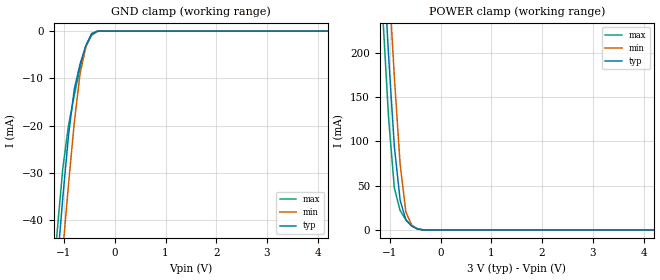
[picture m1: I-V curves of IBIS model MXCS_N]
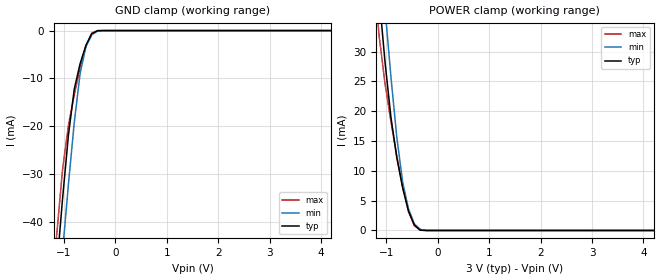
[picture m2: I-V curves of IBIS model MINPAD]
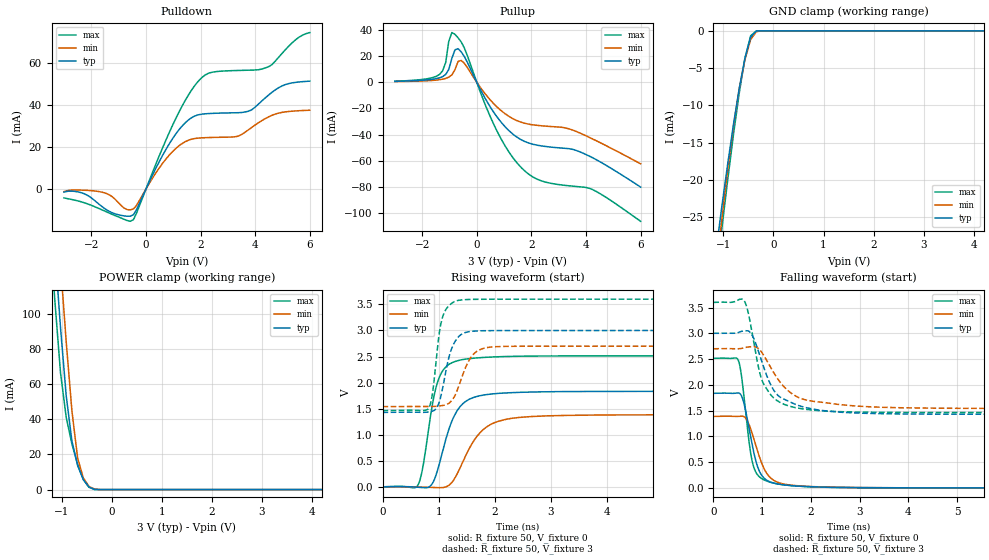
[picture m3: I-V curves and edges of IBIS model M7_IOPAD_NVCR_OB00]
| Created by SiliconSmart  O-2018.09-SP2-3
[IBIS Ver]   4.0
[File Name]   as3204wa_rev1p4.ibs
[File Rev]   1.4
[Date]   Thursday Mar 21 2024
|[Source]   Avalanche Team
|[Notes]   Generated IBIS models from Silicon Smart
|[Rev 1.0]  Initial Release based on extracted netlist
|   Characterization
|[Rev 1.1]  Update the drive strength table for 3V
|[Rev 1.2]  Recharacterization of MIOPAD with Hspice run in high accuracy mode
|[Rev 1.3]  Recharacterization with Hspice to align with datasheet parameter
|[Rev 1.4]  Update the pin to the package pinout assignment
|[Disclaimer]   THE MODEL LIBRARIES ARE PROVIDED AS IS.
|[Copyright]   Copyright 2019, Avalanche Technology., All Rights Reserved
[Component]   AS30xx204_WSON
[Manufacturer] Avalanche Technology
| CONTENT :
| This file contains IBIS MODEL for PSRAM device
| AS3001204 AS3004204 AS3008204 AS3016204
| USAGE :
| The models are derived for the 2.7V to 3.6V I/O Operation.
| Temperatures for model generation: typ: 25, max: -40, min: 105
| Voltages : typ: 3.0V, min: 2.7V, max: 3.6V
| PACKAGES SUPPORTED :
| 8-pad WSON (5.0mm x 6.0mm)
| VERIFICATION
| Errors  : 0
| Warnings: 30
| All warnings due to non-monotonic data:
[Package]
|variable   typ   min   max
R_pkg   8.90E-04   8.89E-04  8.91E-04
L_pkg   1.185E-09  1.18E-09  1.19E-09
C_pkg   2.30E-13   2.21E-13  2.39E-13
[Pin]   signal_name   model_name   R_pin   L_pin   C_pin
1   CS#   MXCS_N   1.05E-01  1.35E-09  9.16E-14
2   SO   MIOPAD   1.05E-01  1.35E-09  9.16E-14
3   WP#   MIOPAD   1.05E-01  1.35E-09  9.16E-14
5   SI   MIOPAD   3.75E-02  3.89E-10  4.24E-14
6   CLK   MINPAD   3.75E-02  3.89E-10  4.24E-14
7   IO_3   MIOPAD   3.75E-02  3.89E-10  4.24E-14
4   VSS   GND   NA   NA   NA
8   VCC   POWER   NA   NA   NA
[Model Selector] MIOPAD
| Model Description
M0_IOPAD_NVCR_OB07   15 Ohms drv strength
M1_IOPAD_NVCR_OB06   20 Ohms drv strength
M2_IOPAD_NVCR_OB05   40 Ohms drv strength
M3_IOPAD_NVCR_OB04   35 Ohms drv strength
M4_IOPAD_NVCR_OB03   45 Ohms drv strength
M5_IOPAD_NVCR_OB02   60 Ohms drv strength
M6_IOPAD_NVCR_OB01   75 Ohms drv strength
M7_IOPAD_NVCR_OB00   35 Ohms drv strength
| Models and submodels in the file (10): MXCS_N (Input), MINPAD (Input), M7_IOPAD_NVCR_OB00 (I/O), M3_IOPAD_NVCR_OB04 (I/O), M5_IOPAD_NVCR_OB02 (I/O), M1_IOPAD_NVCR_OB06 (I/O), M6_IOPAD_NVCR_OB01 (I/O), M2_IOPAD_NVCR_OB05 (I/O), M4_IOPAD_NVCR_OB03 (I/O), M0_IOPAD_NVCR_OB07 (I/O)
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| XCS_N
[Model] MXCS_N
Model_type Input
Enable   Active-High
Vinl  =  0.9
Vinh  =  2.1
| Capacitance  typ   min   max
C_comp   3.070316e-12   2.808436e-12   3.350457e-12
| Variables   typ   min   max
[GND Clamp Reference]   0   0   0
[POWER Clamp Reference]   3   2.7   3.6
[Pulldown Reference]   0   0   0
[Pullup Reference]   3   2.7   3.6
[Temperature Range]   25   105   -40
[Voltage Range]   3   2.7   3.6
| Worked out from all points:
|   GND clamp passes 1 mA (typ) near -0.47 V on its own axis
|   POWER clamp passes 1 mA (typ) near -0.45 V on its own axis
[GND Clamp]
| Voltage   I(typ)   I(min)   I(max)
-3V       -315.1mA   -321.8mA   -312.6mA
-1.138V   -50.1mA    -61.4mA    -42.93mA
-1.024V   -35.38mA   -46.59mA   -29.17mA
-910.3mV  -22.01mA   -32.38mA   -19.91mA
-796.6mV  -12.29mA   -19.34mA   -13.52mA
-682.8mV  -6.93mA    -8.967mA   -7.783mA
-569mV    -3.073mA   -3.363mA   -3.169mA
-455.2mV  -632.4uA   -876.6uA   -499.8uA
-341.4mV  -24.5uA    -77.16uA   -7.616uA
-227.6mV  -421.5nA   -3.518uA   -35.99nA
6V        0A         0A         0A
[POWER Clamp]
| Voltage   I(typ)   I(min)   I(max)
-3V       2.46A      2.545A     2.395A
-1.138V   315.5mA    408mA      242.2mA
-1.024V   197.2mA    287.4mA    127mA
-910.3mV  94.22mA    172.8mA    47.4mA
-796.6mV  33.73mA    74.33mA    21.95mA
-682.8mV  11.27mA    20.05mA    11.43mA
-569mV    4.378mA    5.6mA      4.484mA
-455.2mV  1.088mA    1.361mA    987.1uA
-227.6mV  835.3nA    9.424uA    241.1nA
6V        0A         0A         0A
| INPAD
[Model] MINPAD
Model_type Input
Enable   Active-High
Vinl  =  0.9
Vinh  =  2.1
| Capacitance  typ   min   max
C_comp   2.706389e-12   2.515315e-12   2.914212e-12
| Variables   typ   min   max
[GND Clamp Reference]   0   0   0
[POWER Clamp Reference]   3   2.7   3.6
[Pulldown Reference]   0   0   0
[Pullup Reference]   3   2.7   3.6
[Temperature Range]   25   105   -40
[Voltage Range]   3   2.7   3.6
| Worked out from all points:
|   GND clamp passes 1 mA (typ) near -0.47 V on its own axis
|   POWER clamp passes 1 mA (typ) near -0.46 V on its own axis
[GND Clamp]
| Voltage   I(typ)   I(min)   I(max)
-3V       -312.9mA   -319.5mA   -311mA
-1.138V   -49.77mA   -60.97mA   -42.7mA
-1.024V   -35.15mA   -46.28mA   -29.02mA
-910.3mV  -21.89mA   -32.17mA   -19.81mA
-796.6mV  -12.24mA   -19.23mA   -13.45mA
-682.8mV  -6.904mA   -8.93mA    -7.747mA
-569mV    -3.064mA   -3.355mA   -3.158mA
-455.2mV  -631.5uA   -875.4uA   -499.1uA
-341.4mV  -24.5uA    -77.14uA   -7.616uA
-227.6mV  -421.5nA   -3.518uA   -35.99nA
6V        0A         0A         0A
[POWER Clamp]
| Voltage   I(typ)   I(min)   I(max)
-3V       249.7mA    259.7mA    242mA
-1.252V   50.97mA    61.19mA    43.36mA
-1.138V   39.14mA    48.99mA    32.5mA
-1.024V   28.15mA    37.13mA    24.58mA
-910.3mV  19.01mA    25.79mA    18.3mA
-796.6mV  12.24mA    15.66mA    12.48mA
-682.8mV  7.193mA    8.146mA    7.285mA
-569mV    3.26mA     3.629mA    3.179mA
-455.2mV  915uA      1.117mA    809.1uA
-341.4mV  55.3uA     196.8uA    44.86uA
-113.8mV  7.997nA    354.9nA    881.5pA
6V        0A         0A         0A
[Model] M7_IOPAD_NVCR_OB00
Model_type I/O
Enable   Active-High
Vinl  =  0.9
Vinh  =  2.1
Vmeas =  1.5
Cref  =  30e-12
| Capacitance  typ   min   max
C_comp   3.872127e-12   3.590660e-12   4.176448e-12
| Variables   typ   min   max
[GND Clamp Reference]   0   0   0
[POWER Clamp Reference]   3   2.7   3.6
[Pulldown Reference]   0   0   0
[Pullup Reference]   3   2.7   3.6
[Temperature Range]   25   105   -40
[Voltage Range]   3   2.7   3.6
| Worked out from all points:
|   slope of the pulldown table from 0 to 0.45 V, typ, clamps not added: 37.1 ohm
|   slope of the pullup table from 0 to 0.45 V, typ, clamps not added: 25.9 ohm
|   GND clamp passes 1 mA (typ) near -0.46 V on its own axis
|   POWER clamp passes 1 mA (typ) near -0.42 V on its own axis
|   falling waveform, R_fixture 50, V_fixture 0: 20-80 % time 256ps typ, 321ps min, 201ps max; typ from 1.83 V to 0 V
|   falling waveform, R_fixture 50, V_fixture 3: 20-80 % time 490ps typ, 612ps min, 350ps max; typ from 3 V to 1.43 V
|   rising waveform, R_fixture 50, V_fixture 0: 20-80 % time 339ps typ, 461ps min, 243ps max; typ from 0 V to 1.83 V
|   rising waveform, R_fixture 50, V_fixture 3: 20-80 % time 204ps typ, 266ps min, 147ps max; typ from 1.43 V to 3 V
[GND Clamp]
| Voltage   I(typ)   I(min)   I(max)
-3V       -145.9mA   -151.9mA   -144.2mA
-1.138V   -29.07mA   -31.55mA   -32.68mA
-1.024V   -23.24mA   -24.83mA   -26.15mA
-910.3mV  -17.69mA   -18.46mA   -19.83mA
-796.6mV  -12.47mA   -12.67mA   -13.82mA
-682.8mV  -7.718mA   -7.754mA   -8.316mA
-569mV    -3.663mA   -3.867mA   -3.675mA
-455.2mV  -839.2uA   -1.152mA   -666.1uA
-341.4mV  -35.63uA   -111.1uA   -11.17uA
-113.8mV  -8.642nA   -188.3nA   -1.888nA
6V        0A         0A         0A
[POWER Clamp]
| Voltage   I(typ)   I(min)   I(max)
-3V       949.8mA    984.2mA    923.5mA
-1.252V   183.6mA    221.4mA    154mA
-1.138V   136.7mA    174.2mA    107.6mA
-1.024V   92.09mA    128.1mA    66.35mA
-910.3mV  53.33mA    83.97mA    41.06mA
-796.6mV  27.72mA    44.75mA    25.94mA
-682.8mV  13.75mA    18.06mA    14.29mA
-569mV    5.664mA    6.605mA    5.738mA
-455.2mV  1.446mA    1.789mA    1.305mA
-341.4mV  77.09uA    287.6uA    62.73uA
-227.6mV  1.148uA    12.92uA    332nA
6V        0A         0A         0A
[Pulldown]
| Voltage   I(typ)   I(min)   I(max)
-3V       -1.433mA   -1.188mA   -4.157mA
-2.276V   -2.108mA   -517.7uA   -6.425mA
-1.593V   -8.473mA   -1.507mA   -9.973mA
-455.2mV  -12.21mA   -9.42mA    -14.49mA
931mV     23.15mA    17.28mA    29.13mA
1.448V    31.69mA    22.63mA    42.45mA
1.966V    35.52mA    24.35mA    52.07mA
2.483V    36.1mA     24.62mA    55.8mA
3.745V    37.06mA    28.17mA    56.63mA
4.49V     44.79mA    34.41mA    58.29mA
5.11V     49.81mA    36.8mA     66.46mA
6V        51.42mA    37.57mA    74.56mA
[Pullup]
| Voltage   I(typ)   I(min)   I(max)
-3V       653.5uA    487.7uA    766.8uA
-1.366V   3.311mA    1.902mA    5.899mA
-1.138V   5.906mA    2.886mA    14.98mA
-1.024V   9.73mA     3.87mA     31.24mA
-910.3mV  18.3mA     5.605mA    37.88mA
-796.6mV  24.73mA    9.674mA    36.53mA
-569mV    23.14mA    16.61mA    30.71mA
620.7mV   -22.92mA   -16.38mA   -32.1mA
1.655V    -44.22mA   -30.74mA   -65.72mA
2.379V    -48.66mA   -33.29mA   -75.39mA
3.745V    -52.9mA    -38.5mA    -79.8mA
6V        -80.07mA   -62.32mA   -106.2mA
[Ramp]
dV/dt_r   1.10101/0.339017n  0.831927/0.461224n  1.50845/0.242789n
dV/dt_f   0.94313/0.490001n  0.695697/0.612195n  1.28285/0.34977n
R_load = 50
[Falling Waveform]
R_fixture = 50
V_fixture = 0
V_fixture_min = 0
V_fixture_max = 0
| Time   V(typ)   V(min)   V(max)
0s        1.835V     1.387V     2.514V
508.1ps   1.842V     1.388V     2.484V
563ps     1.81V      1.393V     2.266V
628.4ps   1.639V     1.383V     1.772V
754.2ps   1.042V     1.175V     742mV
850.8ps   600.9mV    886.9mV    345.7mV
956.7ps   299.5mV    569.6mV    204.1mV
1.112ns   137.8mV    259.2mV    126.2mV
1.514ns   51.15mV    62.52mV    51.11mV
21.88ns   622.8nV    711.5nV    10.89uV
[Falling Waveform]
R_fixture = 50
V_fixture = 3
V_fixture_min = 2.7
V_fixture_max = 3.6
| Time   V(typ)   V(min)   V(max)
0s        3V         2.7V       3.6V
624.2ps   3.048V     2.717V     3.642V
788.3ps   2.977V     2.741V     3.046V
963.4ps   2.539V     2.667V     2.19V
1.115ns   2.134V     2.441V     1.888V
1.308ns   1.809V     2.134V     1.693V
1.506ns   1.7V       1.909V     1.603V
2.036ns   1.53V      1.682V     1.509V
4.777ns   1.43V      1.545V     1.463V
21.88ns   1.428V     1.54V      1.462V
[Rising Waveform]
R_fixture = 50
V_fixture = 0
V_fixture_min = 0
V_fixture_max = 0
| Time   V(typ)   V(min)   V(max)
0s        414.5nV    452.2nV    10.8uV
619.8ps   -611.3uV   5.242mV    21.45mV
717.4ps   -8.991mV   2.623mV    378.7mV
871ps     45.71mV    -3.239mV   1.477V
1.013ns   453.4mV    -9.161mV   2.11V
1.262ns   1.331V     129.2mV    2.395V
1.571ns   1.696V     791.7mV    2.465V
2.006ns   1.791V     1.241V     2.495V
2.928ns   1.827V     1.365V     2.512V
21.88ns   1.835V     1.387V     2.514V
[Rising Waveform]
R_fixture = 50
V_fixture = 3
V_fixture_min = 2.7
V_fixture_max = 3.6
| Time   V(typ)   V(min)   V(max)
0s        1.428V     1.54V      1.462V
810.7ps   1.438V     1.544V     1.497V
887.5ps   1.456V     1.544V     1.779V
1.003ns   1.607V     1.552V     2.894V
1.068ns   1.883V     1.562V     3.253V
1.21ns    2.592V     1.633V     3.502V
1.401ns   2.923V     2.069V     3.585V
1.668ns   2.99V      2.593V     3.597V
2.078ns   2.998V     2.692V     3.599V
21.88ns   3V         2.7V       3.6V
